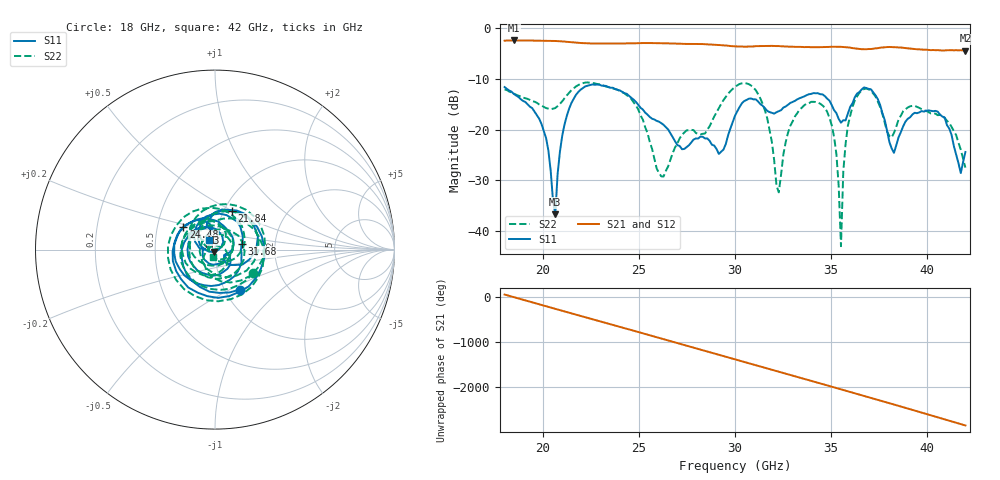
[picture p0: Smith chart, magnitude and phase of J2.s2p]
!Agilent Technologies,N5230A,US43500212,A.07.50.67
!Agilent N5230A: A.07.50.67
!Date: Monday, September 22, 2025 05:42:45
!Correction: S11(Full 2 Port(1,2))
!S21(Full 2 Port(1,2))
!S12(Full 2 Port(1,2))
!S22(Full 2 Port(1,2))
!S2P File: Measurements: S11, S21, S12, S22:
# Hz S  dB  R 50
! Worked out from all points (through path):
!   201 points, 18 GHz to 42 GHz, reference 50 ohm
!   highest |S21| = -2.41 dB at 18.48 GHz (marker M1); lowest = -4.4 dB at 42 GHz (marker M2)
!   lowest |S11| = -36.7 dB at 20.64 GHz (marker M3), VSWR 1.03, Z = 49.6 - j1.38 ohm
!   |S11| at or under -10 dB: start of sweep to end of sweep
!   |S22| runs from -43.0 to -10.7 dB; largest |S21 - S12| = 0.0063
!   S11 on the Smith chart (normalised r, x): 18 GHz: 1.18, -0.56; 21.84 GHz: 1.08, +0.50; 24.48 GHz: 0.68, +0.18; 31.68 GHz: 1.35, +0.09; 42 GHz: 0.94, +0.10
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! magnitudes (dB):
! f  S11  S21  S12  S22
! 18 GHz  -11.6  -2.4  -2.4  -12.1
! 18.48 GHz  -13.0  -2.4  -2.4  -12.9
! 19.92 GHz  -18.9  -2.5  -2.5  -15.2
! 20.64 GHz  -36.7  -2.5  -2.5  -15.8
! 21 GHz  -21.3  -2.6  -2.6  -14.4
! 21.84 GHz  -12.6  -2.9  -2.9  -11.2
! 22.08 GHz  -11.8  -2.9  -2.9  -10.9
! 24.48 GHz  -13.4  -3.0  -3.0  -13.6
! 26.04 GHz  -18.5  -2.9  -2.9  -28.6
! 29.16 GHz  -24.8  -3.3  -3.3  -15.8
! 30 GHz  -17.3  -3.6  -3.6  -11.6
! 31.68 GHz  -16.3  -3.5  -3.5  -17.8
! 32.28 GHz  -16.4  -3.5  -3.5  -32.4
! 32.88 GHz  -14.7  -3.6  -3.6  -19.3
! 34.08 GHz  -12.8  -3.7  -3.7  -14.5
! 35.16 GHz  -16.2  -3.7  -3.6  -21.5
! 35.52 GHz  -18.6  -3.7  -3.7  -43.0
! 35.76 GHz  -18.2  -3.7  -3.7  -22.8
! 36.24 GHz  -13.6  -4.0  -4.0  -14.3
! 38.04 GHz  -22.4  -3.7  -3.7  -21.3
! 40.68 GHz  -17.1  -4.4  -4.3  -17.1
! 42 GHz  -24.4  -4.4  -4.4  -27.5
